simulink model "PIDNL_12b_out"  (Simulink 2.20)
settings: Solver=VariableStepDiscrete  StartTime=0.0  StopTime=40.0  RelTol=1e-3  AbsTol=1e-6
undefined symbols (not defined in the file or in its folder): pidin
libraries: simulink x6, Puma x3

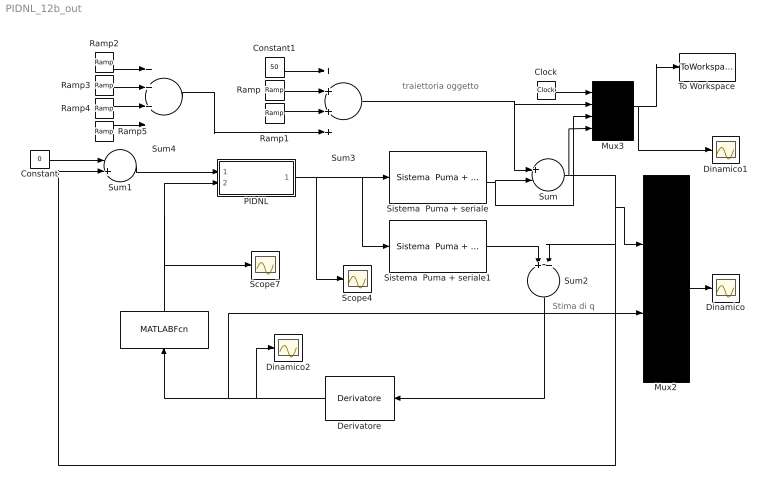
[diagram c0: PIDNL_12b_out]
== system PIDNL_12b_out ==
  note: Stima di q
  note: traiettoria oggetto
  " " : MATLABFcn  Orientation=up  MATLABFcn=1  OutputWidth=-1
  Clock : Clock
  Constant : Constant  Value=0
  Constant1 : Constant  Value=50
  Derivatore : Puma/Derivatore  Orientation=left  Td=0.13  T=0.033  N=10
  Dinamico : Scope
  Dinamico1 : Scope
  Dinamico2 : Scope
  Mux2 : Mux  Inputs=2
  Mux3 : Mux  Inputs=4
  PIDNL : Subsystem
  Ramp : simulink/Sources/Ramp  slope=-50  start=10  X0=0
  Ramp1 : simulink/Sources/Ramp  slope=+50  start=25  X0=0
  Ramp2 : simulink/Sources/Ramp  slope=-50  start=30  X0=0
  Ramp3 : simulink/Sources/Ramp  slope=50  start=31  X0=0
  Ramp4 : simulink/Sources/Ramp  slope=50  start=35  X0=0
  Ramp5 : simulink/Sources/Ramp  slope=-50  start=36  X0=0
  Scope4 : Scope
  Scope7 : Scope
  Sistema  Puma + seriale : Puma/Sistema  Puma + seriale  Ts=.260
  Sistema  Puma + seriale1 : Puma/Sistema  Puma + seriale  Ts=.260
  Sum : Sum  Inputs=+-
  Sum1 : Sum  Inputs=-+
  Sum2 : Sum  Orientation=down  Inputs=++
  Sum3 : Sum  Inputs=++++
  Sum4 : Sum  Inputs=++++
  To Workspace : ToWorkspace  VariableName=int  SampleTime=-1
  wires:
  Sistema  Puma + seriale1/1 -> Sum2/1
  Mux2/1 -> Dinamico/1
  Sum2/1 -> Derivatore/1
  Constant1/1 -> Sum3/1
  Sum1/1 -> PIDNL/1(In1)
  Constant/1 -> Sum1/1
  PIDNL/1(Out1) -> Sistema  Puma + seriale/1, Sistema  Puma + seriale1/1, Scope4/1
  Ramp/1 -> Sum3/2
  Ramp1/1 -> Sum3/3
  " "/1 -> PIDNL/2(In2), Scope7/1
  Mux3/1 -> To Workspace/1, Dinamico1/1
  Sistema  Puma + seriale/1 -> Sum/2, Mux3/3
  Sum3/1 -> Sum/1, Mux3/2
  Clock/1 -> Mux3/1
  Sum/1 -> Sum2/2, Sum1/2, Mux2/1, Mux3/4
  Derivatore/1 -> Dinamico2/1, " "/1, Mux2/2
  Ramp5/1 -> Sum4/4
  Ramp4/1 -> Sum4/3
  Ramp3/1 -> Sum4/2
  Ramp2/1 -> Sum4/1
  Sum4/1 -> Sum3/4

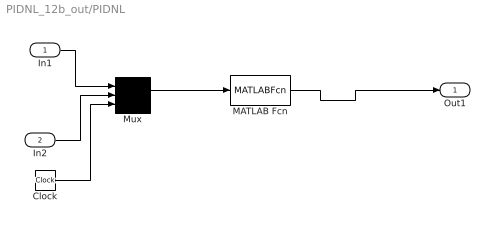
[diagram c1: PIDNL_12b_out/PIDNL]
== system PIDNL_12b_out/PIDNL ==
  In1 : Inport  Port=1  PortWidth=-1  SampleTime=-1
  In2 : Inport  Port=2  PortWidth=-1  SampleTime=-1
  Clock : Clock
  MATLAB Fcn : MATLABFcn  MATLABFcn=pidin(u(1),u(2),u(3))  OutputWidth=1
  Mux : Mux  Inputs=3
  Out1 : Outport  Port=1
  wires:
  MATLAB Fcn/1 -> Out1/1
  Mux/1 -> MATLAB Fcn/1
  In1/1 -> Mux/1
  In2/1 -> Mux/2
  Clock/1 -> Mux/3
